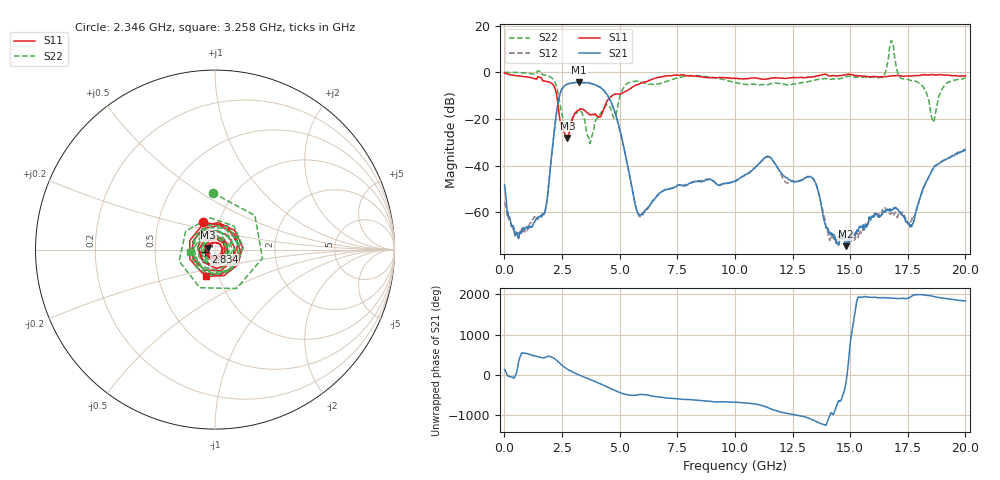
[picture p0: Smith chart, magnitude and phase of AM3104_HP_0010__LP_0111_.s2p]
!Created with skrf (http://scikit-rf.org).
# Hz S RI R 50.0
!freq ReS11 ImS11 ReS21 ImS21 ReS12 ImS12 ReS22 ImS22
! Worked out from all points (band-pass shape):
!   1601 points, 10 MHz to 20 GHz, reference 50 ohm
!   highest |S21| = -4.33 dB at 3.246 GHz (marker M1); lowest = -74.6 dB at 14.8 GHz (marker M2)
!   |S21| within 3 dB of the highest: 2.489 GHz to 4.272 GHz (1.783 GHz wide, 52.8 % of centre)
!   lowest |S11| = -28.2 dB at 2.734 GHz (marker M3), VSWR 1.08, Z = 46.4 + j0.928 ohm
!   |S11| at or under -10 dB: 2.272 GHz to 4.684 GHz (2.412 GHz wide, 69.4 % of centre)
!   |S22| runs from -30.6 to 13.6 dB; largest |S21 - S12| = 0.037
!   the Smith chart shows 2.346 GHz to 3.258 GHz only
!   S11 on the Smith chart (normalised r, x): 2.346 GHz: 0.84, +0.26; 2.834 GHz: 0.90, -0.02; 3.258 GHz: 0.87, -0.27
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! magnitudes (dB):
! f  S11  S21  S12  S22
! 10 MHz  -0.4  -48.3  -55.7  0.0
! 534.7 MHz  -1.5  -68.9  -68.8  -0.1
! 1.697 GHz  -3.8  -60.9  -60.7  -1.1
! 2.346 GHz  -15.6  -12.1  -12.2  -10.0
! 2.734 GHz  -28.2  -5.1  -5.1  -23.9
! 2.834 GHz  -25.0  -4.7  -4.8  -22.4
! 3.246 GHz  -16.3  -4.3  -4.4  -16.8
! 3.258 GHz  -16.1  -4.3  -4.4  -16.9
! 3.346 GHz  -15.8  -4.4  -4.5  -17.0
! 3.708 GHz  -18.3  -4.7  -4.7  -30.6
! 4.645 GHz  -10.3  -13.1  -13.2  -16.7
! 5.832 GHz  -5.1  -60.8  -61.6  -3.9
! 6.682 GHz  -2.2  -52.5  -52.3  -5.0
! 10.01 GHz  -2.7  -46.8  -46.8  -4.5
! 11.43 GHz  -2.8  -36.0  -36.3  -5.4
! 13.34 GHz  -2.1  -45.2  -45.1  -3.7
! 14.05 GHz  -1.4  -67.5  -69.9  -3.0
! 14.8 GHz  -1.1  -74.6  -71.0  -2.0
! 16.68 GHz  -1.7  -59.3  -59.6  7.2
! 17.68 GHz  -1.7  -65.6  -63.3  -3.7
! 18.6 GHz  -1.1  -41.4  -41.5  -21.3
! 20 GHz  -1.5  -33.4  -32.9  -2.6
